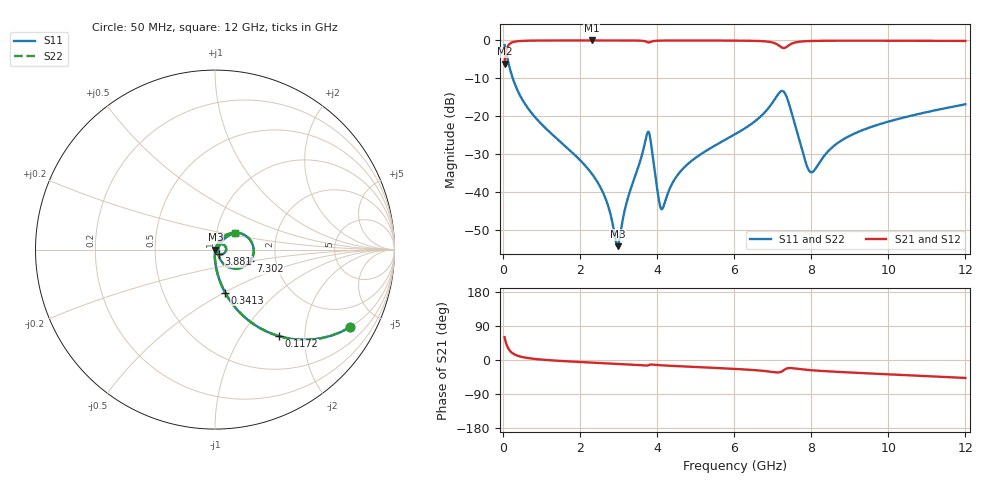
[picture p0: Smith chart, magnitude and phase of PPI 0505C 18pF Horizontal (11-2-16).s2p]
# MHz S MA R 50
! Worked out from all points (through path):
!   1601 points, 50 MHz to 12 GHz, reference 50 ohm
!   highest |S21| = -0.02 dB at 2.306 GHz (marker M1); lowest = -6.1 dB at 50 MHz (marker M2)
!   group delay of S21, straight-line fit = 12.5 ps
!   lowest |S11| = -54.3 dB at 2.978 GHz (marker M3), VSWR 1.00, Z = 50.2 - j0.0395 ohm
!   |S11| at or under -10 dB: 261.7 MHz to end of sweep
!   |S22| runs from -54.3 to -1.2 dB; largest |S21 - S12| = 0
!   S11 on the Smith chart (normalised r, x): 50 MHz: 0.99, -3.49; 117.2 MHz: 0.99, -1.49; 341.3 MHz: 0.99, -0.51; 3.881 GHz: 1.05, -0.05; 7.302 GHz: 1.48, -0.20; 12 GHz: 1.22, +0.23
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50  0.8689 -29.8  0.4948 60.2  0.4948 60.2  0.8689 -29.8
117.2188  0.5989 -53.6  0.8005 36.4  0.8005 36.4  0.5989 -53.6
341.2812  0.2465 -76.7  0.9685 13.1  0.9685 13.1  0.2465 -76.7
849.1562  0.09597 -86.8  0.9944 2.6  0.9944 2.6  0.09597 -86.8
2044.156  0.02522 -92.4  0.9982 -5.5  0.9982 -5.5  0.02522 -92.4
2305.562  0.01763 -92.0  0.9982 -6.8  0.9982 -6.8  0.01763 -92.0
2679  0.007956 -86.5  0.9981 -8.6  0.9981 -8.6  0.007956 -86.5
2977.75  0.001936 -11.7  0.9979 -10.1  0.9979 -10.1  0.001936 -11.7
3732.094  0.05544 28.8  0.9589 -14.8  0.9589 -14.8  0.05544 28.8
3799.312  0.05976 -11.3  0.94 -12.9  0.94 -12.9  0.05976 -11.3
3881.469  0.03254 -46.1  0.9726 -12.1  0.9726 -12.1  0.03254 -46.1
4038.312  0.008625 -36.7  0.9918 -13.4  0.9918 -13.4  0.008625 -36.7
4142.875  0.00604 14.3  0.9944 -14.2  0.9944 -14.2  0.00604 14.3
4703.031  0.02102 64.8  0.9965 -17.0  0.9965 -17.0  0.02102 64.8
6025  0.05785 61.7  0.9931 -23.5  0.9931 -23.5  0.05785 61.7
7033.281  0.1607 35.5  0.927 -32.0  0.927 -32.0  0.1607 35.5
7302.156  0.2073 -18.0  0.7938 -26.0  0.7938 -26.0  0.2073 -18.0
7869.781  0.02357 -40.7  0.9767 -25.9  0.9767 -25.9  0.02357 -40.7
8019.156  0.01825 -1.8  0.983 -27.1  0.983 -27.1  0.01825 -1.8
8766.031  0.04718 49.3  0.991 -31.7  0.991 -31.7  0.04718 49.3
10013.31  0.08526 48.7  0.9906 -37.9  0.9906 -37.9  0.08526 48.7
12000  0.1437 40.7  0.984 -47.4  0.984 -47.4  0.1437 40.7
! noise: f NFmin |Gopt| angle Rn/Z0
50  0.0003906  0.8669  1.215  0.0006306
1372  0.003976  0.6735  4.896  0.002342
2701  0.006844  0.636  9.194  0.00352
4031  0.0182  0.779  13.62  0.01663
5360  0.0133  0.6331  17.8  0.00666
6682  0.03161  0.7908  22.2  0.03001
8012  0.03628  0.7843  26.65  0.03275
9341  0.02323  0.6425  30.51  0.01148
1.067e+04  0.02284  0.6005  34.23  0.009679
1.2e+04  0.02419  0.5857  37.87  0.009613
